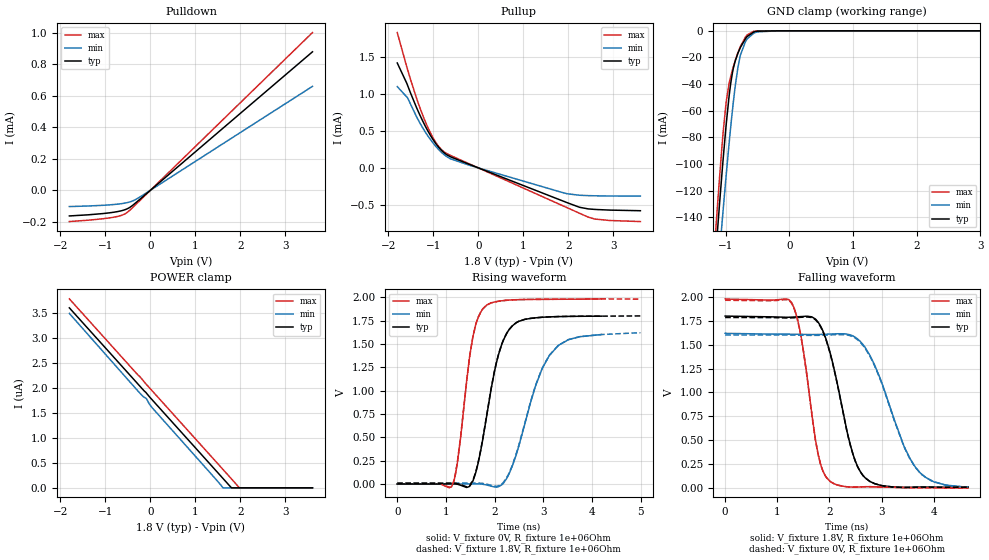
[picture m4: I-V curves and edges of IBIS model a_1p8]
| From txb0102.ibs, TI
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|   a_1p8 Model
[Model]   a_1p8
Model_type   I/O
Polarity   Non-Inverting
Enable   Active-High
Vinl = 0.63
Vinh = 1.17
Vmeas = 0.9
Vref = 0
Cref = 2pF
Rref = 1e6
|   typ   min   max
|   (nom PVT)   (fast PVT)   (slow PVT)
C_comp   3.930e-12   3.869e-12   3.930e-12
[Model spec]
|subparameter
Vinl   0.63   0.567   0.693
Vinh   1.17   1.053   1.287
| Where nom  PVT is Nominal Process, 1.8V, 27C
|   Fast PVT is Strong Process,  1.98V, -40C
|   Slow PVT is Weak Process,   1.62V, 125C
[Voltage Range]   1.8   1.62   1.98
|Junction Temperature
[Temperature Range]   27   125   -40
[Pullup Reference]   1.8   1.62   1.98
[Pulldown Reference]   0   0   0
[Power Clamp Reference]   1.8   1.62   1.98
[GND Clamp Reference]   0   0   0
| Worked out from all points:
|   slope of the pulldown table from 0 to 0.27 V, typ, clamps not added: 4.09 kohm
|   slope of the pullup table from 0 to 0.27 V, typ, clamps not added: 4.18 kohm
|   GND clamp passes 1 mA (typ) near -0.56 V on its own axis
|   falling waveform, V_fixture 1.8V, R_fixture 1e+06Ohm: 20-80 % time 446ps typ, 665ps min, 313ps max; typ from 1.8 V to 0.007 V
|   rising waveform, V_fixture 0V, R_fixture 1e+06Ohm: 20-80 % time 396ps typ, 576ps min, 281ps max; typ from 0 V to 1.8 V
|   rising waveform, V_fixture 1.8V, R_fixture 1e+06Ohm: 20-80 % time 397ps typ, 589ps min, 280ps max; typ from 0.007 V to 1.8 V
|   falling waveform, V_fixture 0V, R_fixture 1e+06Ohm: 20-80 % time 443ps typ, 658ps min, 311ps max; typ from 1.78 V to 0.007 V
[Pulldown]
|   Voltage   I(typ)   I(min)   I(max)
-1.8V     -163uA     -103.4uA   -198.6uA
-812mV    -139.3uA   -90.36uA   -171uA
-621mV    -128.3uA   -83.98uA   -156.9uA
-497.5mV  -115.1uA   -77.11uA   -136.7uA
-367.2mV  -89.48uA   -64.17uA   -102.3uA
-180mV    -44.06uA   -33.02uA   -50.15uA
3.6V      879.5uA    660.1uA    1.002mA
[GND Clamp]
|   Voltage   I(typ)   I(min)   I(max)
-1.8V     -624.1mA   -621.9mA   -639.9mA
-1.206V   -199.4mA   -231.9mA   -183.8mA
-1.141V   -157.4mA   -192.7mA   -138.9mA
-1.095V   -128.6mA   -165.6mA   -108.8mA
-1.057V   -105.5mA   -143.4mA   -85.31mA
-990mV    -68.89mA   -106.7mA   -52.45mA
-894.6mV  -31.48mA   -59.58mA   -29.35mA
-780.3mV  -13.62mA   -20.51mA   -12.96mA
-662.4mV  -4.253mA   -6.03mA    -3.026mA
-505.6mV  -290.2uA   -812.9uA   -74.19uA
-180mV    -201.7nA   -1.304uA   -180.2nA
3.6V      0A         0A         0A
[Pullup]
|   Voltage   I(typ)   I(min)   I(max)
-1.8V     1.421mA    1.101mA    1.833mA
-1.576V   1.127mA    952.6uA    1.344mA
-1.376V   822.4uA    697.9uA    951.3uA
-1.236V   635.8uA    543.1uA    715.2uA
-1.009V   386.9uA    340.3uA    411.6uA
-881.3mV  279.7uA    249.2uA    291uA
-755.1mV  202.1uA    177.6uA    215uA
-180mV    43.04uA    32.24uA    49.34uA
1.9V      -453.9uA   -339.2uA   -519.8uA
2.25V     -534.3uA   -370.8uA   -615.3uA
2.587V    -563uA     -378.3uA   -693.5uA
3.6V      -580.5uA   -382.5uA   -727.4uA
[POWER Clamp]
|   Voltage   I(typ)   I(min)   I(max)
-1.8V     3.601uA    3.489uA    3.78uA
-245.7mV  2.046uA    1.907uA    2.237uA
-162.2mV  1.963uA    1.828uA    2.147uA
-90.9mV   1.898uA    1.785uA    2.071uA
-21.24mV  1.822uA    1.674uA    2.001uA
41.94mV   1.758uA    1.601uA    1.938uA
1.612V    188.3nA    0A         368.3nA
1.802V    0A         0A         178.2nA
1.978V    0A         0A         0A
3.6V      0A         0A         0A
[Ramp]
R_load = 1e+06
|   typ   min   max
dV/dt_r   1.07535/3.92567e-10   0.968384/5.79379e-10   1.18343/2.76587e-10
dV/dt_f   1.07333/4.43867e-10   0.965407/6.63541e-10   1.18085/3.09124e-10
[Falling Waveform]
V_fixture = 1.8V
V_fixture_min = 1.62V
V_fixture_max = 1.98V
R_fixture = 1e+06Ohm
|   Time   V(typ)   V(min)   V(max)
0s        1.8V       1.62V      1.98V
1.276ns   1.789V     1.61V      1.939V
1.462ns   1.795V     1.608V     1.564V
1.784ns   1.735V     1.607V     350.7mV
2.002ns   1.436V     1.611V     73.91mV
2.408ns   435mV      1.602V     9.419mV
2.682ns   107.1mV    1.472V     12.7mV
3.65ns    7.724mV    214.8mV    3.208mV
4.01ns    7.607mV    61.79mV    1.835mV
4.66ns    6.875mV    11.38mV    1.073mV
[Rising Waveform]
V_fixture = 0V
V_fixture_min = 0V
V_fixture_max = 0V
R_fixture = 1e+06Ohm
|   Time   V(typ)   V(min)   V(max)
0s        133nV      45.01uV    28.45nV
1.12ns    2.026mV    -107.9uV   -27.32mV
1.236ns   -2.662mV   -96.31uV   228.1mV
1.55ns    27.09mV    1.443mV    1.564V
1.84ns    735.6mV    -10.81mV   1.917V
2.084ns   1.392V     -27.57mV   1.958V
2.37ns    1.696V     199.6mV    1.972V
2.846ns   1.78V      1.057V     1.977V
3.126ns   1.79V      1.377V     1.978V
4.198ns   1.798V     1.601V     1.983V
[Rising Waveform]
V_fixture = 1.8V
V_fixture_min = 1.62V
V_fixture_max = 1.98V
R_fixture = 1e+06Ohm
|   Time   V(typ)   V(min)   V(max)
0s        7.295mV    8.75mV     7.056mV
1.118ns   9.321mV    8.597mV    -22.11mV
1.234ns   4.851mV    8.606mV    228.2mV
1.55ns    34.29mV    10.15mV    1.567V
1.84ns    742.5mV    -2.083mV   1.917V
2.084ns   1.395V     -18.89mV   1.958V
2.44ns    1.726V     314.9mV    1.974V
2.976ns   1.786V     1.238V     1.978V
3.308ns   1.793V     1.485V     1.979V
4.996ns   1.8V       1.62V      1.98V
[Falling Waveform]
V_fixture = 0V
V_fixture_min = 0V
V_fixture_max = 0V
R_fixture = 1e+06Ohm
|   Time   V(typ)   V(min)   V(max)
0s        1.785V     1.602V     1.966V
1.278ns   1.781V     1.601V     1.931V
1.46ns    1.787V     1.599V     1.563V
1.784ns   1.727V     1.598V     347.2mV
2.002ns   1.429V     1.602V     73.21mV
2.408ns   430.8mV    1.593V     9.324mV
2.68ns    107.2mV    1.465V     12.63mV
3.644ns   8.008mV    216.2mV    3.182mV
3.952ns   8.586mV    73.79mV    1.933mV
4.661ns   6.92mV     11.24mV    1.028mV
